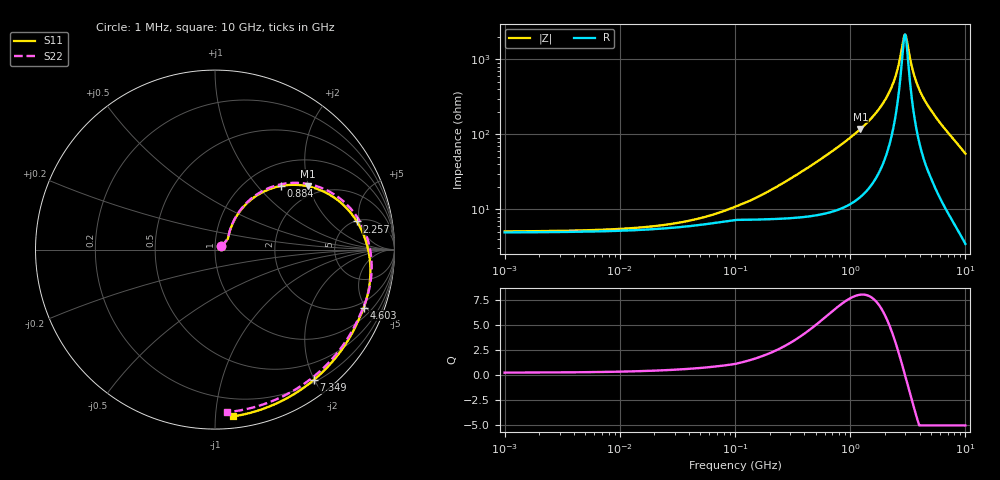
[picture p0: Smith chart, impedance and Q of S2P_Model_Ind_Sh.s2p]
! Created Fri Jun 22 18:17:01 2018
# hz S ma R 50
! 2 Port Network Data from SP2.SP block
! freq  magS11  angS11  magS21  angS21  magS12  angS12  magS22  angS22
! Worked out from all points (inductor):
!   10000 points, 1 MHz to 10 GHz, reference 50 ohm
!   read as 1/Y11, port 2 shorted: L = 12.7 nH near 281 MHz
!   highest Q = 8 at 1.227 GHz (marker M1), where L = 15.2 nH
!   self-resonance near 2.992 GHz
!   S11 on the Smith chart (normalised r, x): 1 MHz: 1.07, +0.04; 884 MHz: 1.40, +1.34; 2.257 GHz: 5.12, +4.58; 4.603 GHz: 1.56, -4.84; 7.349 GHz: 0.23, -1.99; 10 GHz: 0.08, -1.11
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1000000  0.03899 31.2  0.9393 -0.1  0.9393 -0.1  0.03898 31.2
8.1e7  0.08458 38.8  0.9324 -3.8  0.9324 -3.8  0.08459 39.0
1.31e8  0.1113 46.7  0.9289 -6.2  0.9289 -6.2  0.1113 46.9
2.18e8  0.1612 54.9  0.9217 -10.2  0.9217 -10.2  0.1613 55.1
3.15e8  0.2194 57.2  0.91 -14.7  0.91 -14.7  0.2195 57.6
4.27e8  0.2851 56.3  0.8925 -19.6  0.8925 -19.6  0.2853 56.9
5.58e8  0.3576 53.5  0.8676 -25.2  0.8676 -25.2  0.3578 54.2
8.84e8  0.5097 44.1  0.7933 -37.7  0.7933 -37.7  0.5101 45.2
1.227e9  0.6268 34.2  0.7111 -48.9  0.7111 -48.9  0.6276 35.8
1.668e9  0.7273 23.2  0.6161 -60.7  0.6161 -60.7  0.7285 25.3
2.257e9  0.8058 11.2  0.5163 -73.3  0.5163 -73.3  0.8076 13.8
2.759e9  0.8439 2.7  0.4532 -82.2  0.4532 -82.2  0.8459 5.6
3.334e9  0.8693 -5.7  0.4001 -91.1  0.4001 -91.1  0.8711 -2.7
3.947e9  0.8836 -13.6  0.3604 -99.9  0.3604 -99.9  0.8843 -10.7
4.603e9  0.8897 -21.3  0.3327 -109.0  0.3327 -109.0  0.8878 -18.8
5.001e9  0.8903 -25.6  0.3223 -114.5  0.3223 -114.5  0.8857 -23.7
5.822e9  0.8976 -35.2  0.2889 -125.9  0.2889 -125.9  0.8894 -33.9
6.667e9  0.9052 -45.0  0.2544 -137.6  0.2544 -137.6  0.8932 -44.5
7.349e9  0.9113 -52.9  0.2267 -147.1  0.2267 -147.1  0.8963 -53.0
8.334e9  0.9202 -64.4  0.1865 -160.8  0.1865 -160.8  0.9007 -65.2
9.179e9  0.9277 -74.2  0.1521 -172.5  0.1521 -172.5  0.9046 -75.8
1e10  0.9351 -83.8  0.1187 176.1  0.1187 176.1  0.9083 -86.0
